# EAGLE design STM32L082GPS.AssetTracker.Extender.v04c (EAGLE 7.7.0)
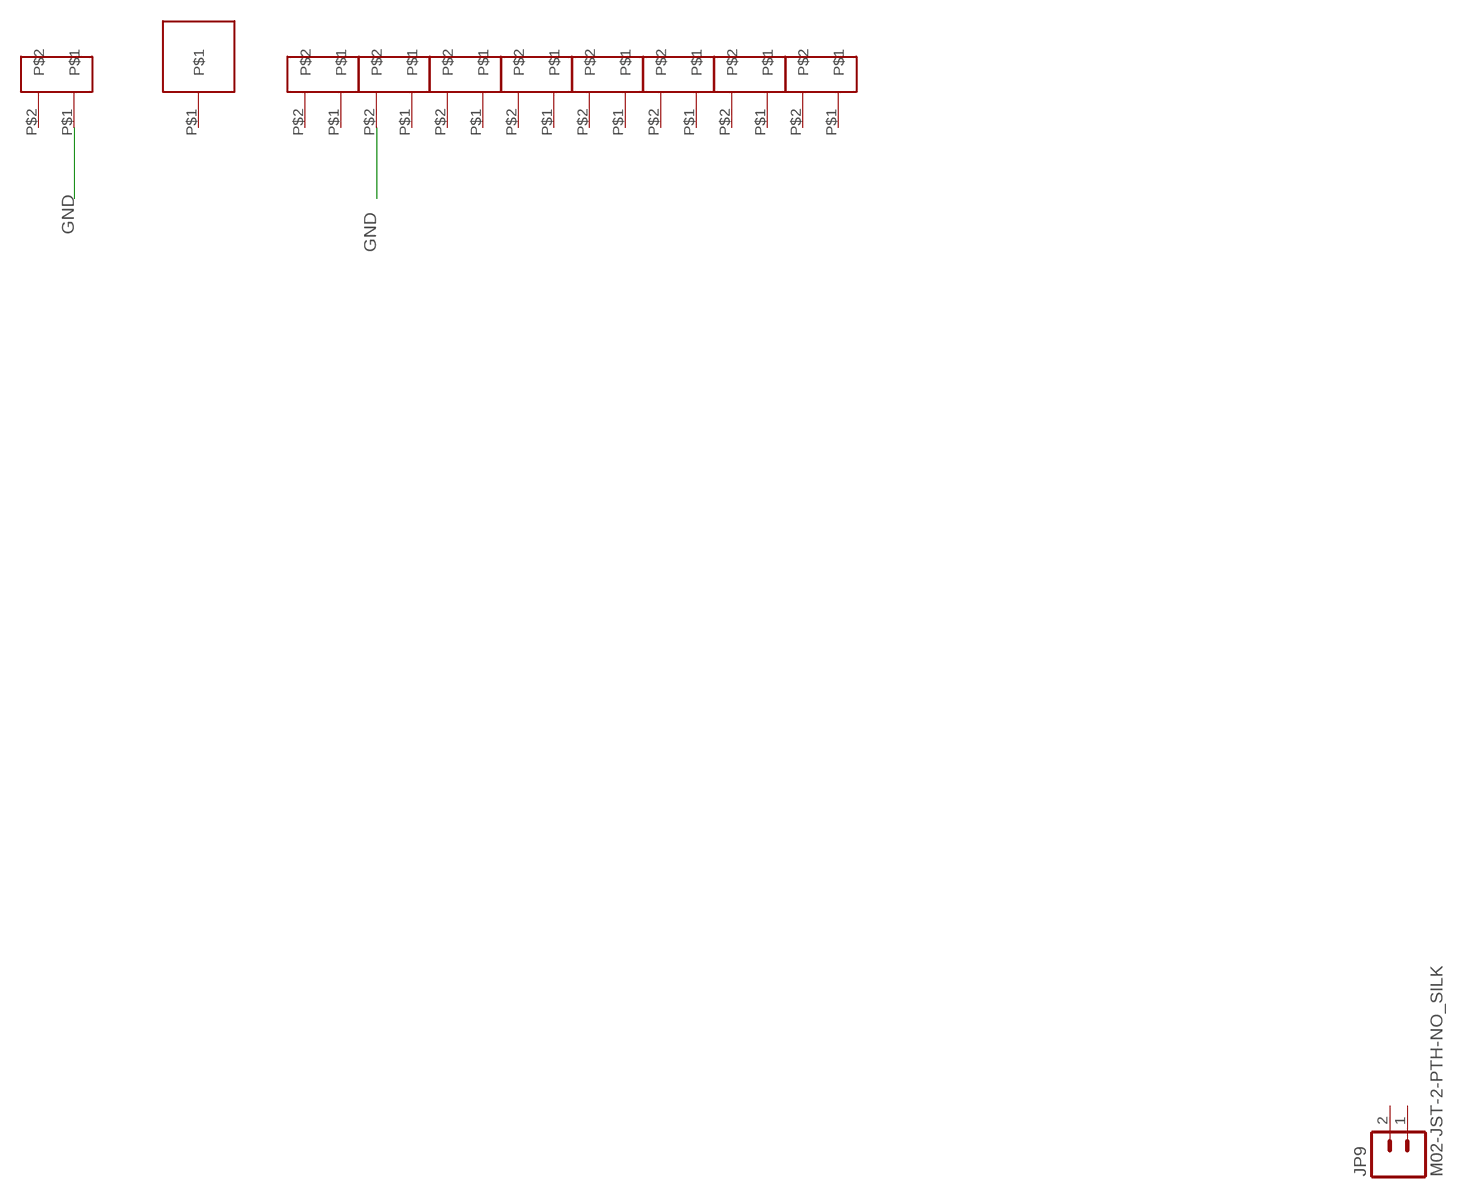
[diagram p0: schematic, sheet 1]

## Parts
JP9  M02-JST-2-PTH-NO_SILK  [JST-2-PTH-NS]
U$1  HN02  [HN02]
U$3  HN02  [HN02]
U$5  HN01  [HN01]
U$11  HN02  [HN02]
U$12  HN02  [HN02]
U$13  HN02  [HN02]
U$14  HN02  [HN02]
U$16  HN02  [HN02]
U$17  HN02  [HN02]
U$36  HN02  [HN02]

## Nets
GND: U$12.P$2 U$36.P$1
Unconnected: JP9.1 JP9.2 U$1.P$1 U$1.P$2 U$3.P$1 U$3.P$2 U$11.P$1 U$11.P$2 U$12.P$1 U$13.P$1 U$13.P$2 U$14.P$1 U$14.P$2 U$16.P$1 U$16.P$2 U$17.P$1 U$17.P$2 U$36.P$2

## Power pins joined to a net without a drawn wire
P$1: U$5.P$1

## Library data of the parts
JP9 = SparkFun-Connectors:M02: Standard 2-pin 0.1" header. Use with
U$1 U$3 U$11-U$14 U$16 U$17 U$36 = Kris:HN02: 0.1 inch header
U$5 = PWSONN6:HN01

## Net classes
1 USB: width 0.254 mm, drill 0.33 mm, clearance 0.159 mm
2 Top GND Pour: clearance 0.762 mm to class 1

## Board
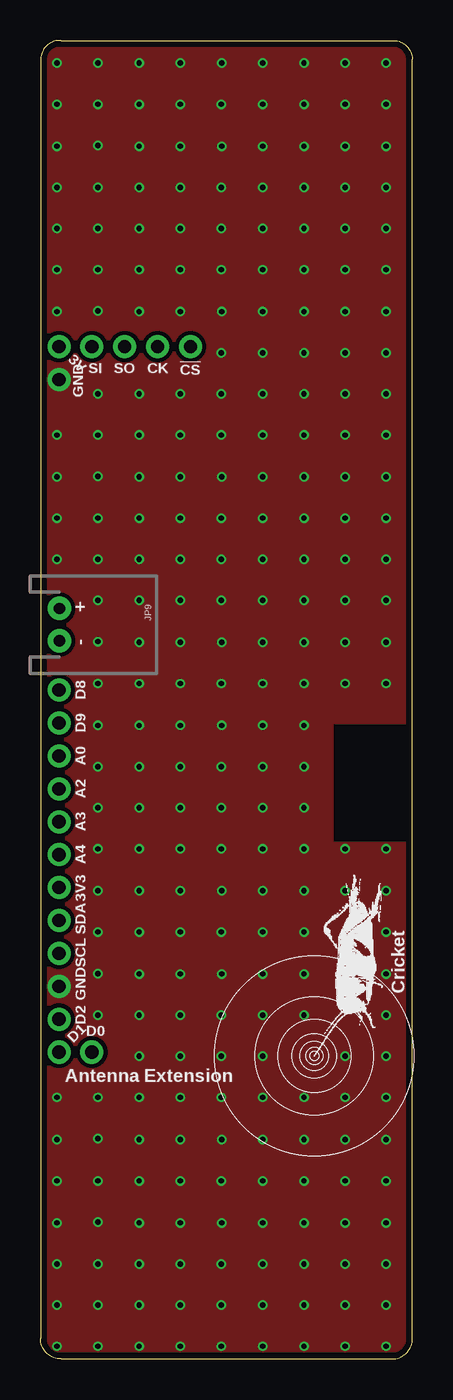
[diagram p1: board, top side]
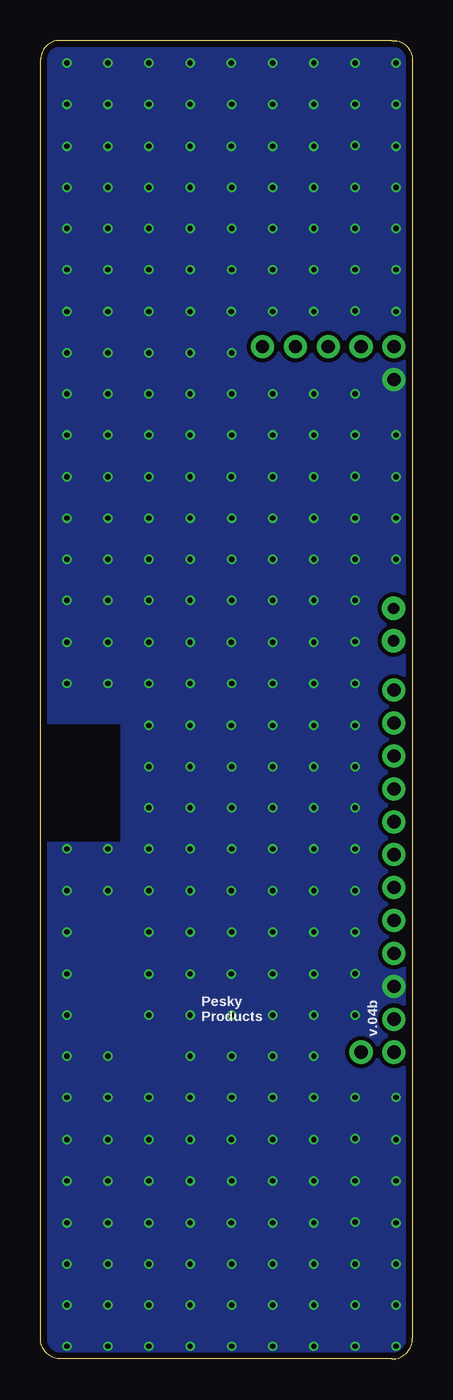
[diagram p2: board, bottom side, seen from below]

Size 22.99 x 81.41 mm. Coordinates in mm from the lower left corner, seen from the top.
Outline: 1.27,0 21.72,0 arc90 22.99,1.27 22.99,80.26 arc90 21.72,81.41 1.27,81.41 arc90 0,80.26 0,1.27 arc90 1.27,0
Copper layers (1*16): Top 0.035559375mm / dielectric 1.6mm / Bottom 0.035559375mm
Design rules "oshpark-2layer *": minimum track width 6mil, minimum drill 10mil, track to track 6mil, track to pad 6mil, pad to pad 6mil, via to via 6mil, smd to smd 6mil, copper to edge 15mil, drill to drill 6mil, minimum pad ring 5mil, minimum via ring 5mil, stop-mask expansion 2.5mil, vias tented up to drill 20mil, thermal gap 10mil

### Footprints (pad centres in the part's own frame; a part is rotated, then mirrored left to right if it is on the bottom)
JST-2-PTH-NS = drill 0.7 pad 1.448: 1 -1,0; 2 1,0
HN02 = drill 0.813 pad 1.422: P$1 0,0; P$2 -2.032,0
HN01 = drill 0.813 pad 1.422: P$1 0,0

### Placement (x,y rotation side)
JP9  1.17,45.34 270 top
U$1  9.27,62.51 0 top
U$3  5.21,62.51 0 top
U$5  1.14,20.98 0 top
U$11  1.14,18.95 180 top
U$12  1.14,25.04 90 top
U$13  1.14,29.11 90 top
U$14  1.14,33.17 90 top
U$16  1.14,41.3 90 top
U$17  1.14,37.24 90 top
U$36  1.14,60.48 270 top

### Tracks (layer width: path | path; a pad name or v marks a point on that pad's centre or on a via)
GND  (via drill 0.33)
  other vias: 1.02,80.01 3.56,80.01 6.1,80.01 8.64,80.01 1.02,77.47 3.56,77.47 6.1,77.47 8.64,77.47 11.18,77.47 3.56,74.93 11.2,80.01 13.74,80.01 16.28,80.01 18.82,80.01 21.36,80.01 13.74,77.47 16.28,77.47 18.82,77.47 21.36,77.47 1.02,74.88 6.1,74.88 8.64,74.88 1.02,72.34 3.56,72.34 6.1,72.34 8.64,72.34 11.18,72.34 1.02,69.8 3.56,69.8 6.1,69.8 8.64,69.8 11.18,69.8 11.2,74.88 13.74,74.88 16.28,74.88 18.82,74.88 21.36,74.88 13.74,72.34 16.28,72.34 18.82,72.34 21.36,72.34 13.74,69.8 16.28,69.8 18.82,69.8 21.36,69.8 1.02,67.26 3.56,67.26 6.1,67.26 8.64,67.26 11.18,67.26 3.56,64.72 13.74,67.26 16.28,67.26 18.82,67.26 21.36,67.26 1.02,64.67 6.1,64.67 8.64,64.67 11.18,62.13 3.56,59.59 6.1,59.59 8.64,59.59 11.18,59.59 11.2,64.67 13.74,64.67 16.28,64.67 18.82,64.67 21.36,64.67 13.74,62.13 16.28,62.13 18.82,62.13 21.36,62.13 13.74,59.59 16.28,59.59 18.82,59.59 21.36,59.59 1.02,57.05 3.56,57.05 6.1,57.05 8.64,57.05 11.18,57.05 3.56,54.51 13.74,57.05 16.28,57.05 18.82,57.05 21.36,57.05 1.02,54.46 6.1,54.46 8.64,54.46 1.02,51.92 3.56,51.92 6.1,51.92 8.64,51.92 11.18,51.92 1.02,49.38 3.56,49.38 6.1,49.38 8.64,49.38 11.18,49.38 11.2,54.46 13.74,54.46 16.28,54.46 18.82,54.46 21.36,54.46 13.74,51.92 16.28,51.92 18.82,51.92 21.36,51.92 13.74,49.38 16.28,49.38 18.82,49.38 21.36,49.38 3.56,46.84 6.1,46.84 8.64,46.84 11.18,46.84 3.56,44.3 13.74,46.84 16.28,46.84 18.82,46.84 21.36,46.84 6.1,44.25 8.64,44.25 11.2,44.25 13.74,44.25 16.28,44.25 18.82,44.25 21.36,44.25 3.56,41.71 6.1,41.71 8.64,41.71 11.18,41.71 3.56,39.12 13.74,41.71 16.28,41.71 18.82,41.71 21.36,41.71 6.1,39.12 8.64,39.12 3.56,36.58 6.1,36.58 8.64,36.58 11.18,36.58 3.56,34.04 6.1,34.04 8.64,34.04 11.18,34.04 11.2,39.12 13.74,39.12 16.28,39.12 13.74,36.58 16.28,36.58 13.74,34.04 16.28,34.04 3.56,31.5 6.1,31.5 8.64,31.5 11.18,31.5 13.74,31.5 16.28,31.5 18.82,31.5 21.36,31.5 6.1,28.91 8.64,28.91 11.2,28.91 13.74,28.91 16.28,28.91 18.82,28.91 21.36,28.91 3.56,28.91 3.56,26.37 6.1,26.37 8.64,26.37 11.18,26.37 3.56,23.8 13.74,26.37 16.28,26.37 21.36,26.37 6.1,23.77 8.64,23.77 3.56,21.23 6.1,21.23 8.64,21.23 11.18,21.23 6.1,18.69 8.64,18.69 11.18,18.69 11.2,23.77 13.74,23.77 16.28,23.77 21.36,23.77 13.74,21.23 16.28,21.23 21.36,21.23 13.74,18.69 18.82,18.69 21.36,18.69 1.02,16.15 3.56,16.15 6.1,16.15 8.64,16.15 11.18,16.15 3.56,13.61 13.74,16.15 16.28,16.15 18.82,16.15 21.36,16.15 1.02,13.54 6.1,13.54 8.64,13.54 1.02,11 3.56,11 6.1,11 8.64,11 11.18,11 3.56,8.46 11.2,13.54 13.74,13.54 16.28,13.54 18.82,13.54 21.36,13.54 13.74,11 16.28,11 18.82,11 21.36,11 1.02,8.41 6.1,8.41 8.64,8.41 1.02,5.87 3.56,5.87 6.1,5.87 8.64,5.87 11.18,5.87 1.02,3.33 3.56,3.33 6.1,3.33 8.64,3.33 11.18,3.33 11.2,8.41 13.74,8.41 16.28,8.41 18.82,8.41 21.36,8.41 13.74,5.87 16.28,5.87 18.82,5.87 21.36,5.87 13.74,3.33 16.28,3.33 18.82,3.33 21.36,3.33 1.02,0.79 3.56,0.79 6.1,0.79 8.64,0.79 11.18,0.79 13.74,0.79 16.28,0.79 18.82,0.79 21.36,0.79
  pour Top (isolate 0.254, no thermals): 0,0 0,81.41 22.99,81.41 23.06,39.29 17.98,39.29 17.98,31.83 22.96,31.83 22.96,0
  pour Bottom (isolate 0.254, no thermals): 0,0 22.99,0 22.99,81.41 0,81.41 -0.03,58.65 0,58.65
N$2
  cutout Bottom (isolate 0.254): 23.04,39.17 18.11,39.17 18.11,31.95 23.04,31.95

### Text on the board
tPlace: 3V | SI | SO | CK | !CS | GND | + | - | D8 | D9 | A0 | A2 | A3 | A4 | 3V3 | SDA | SCL | Cricket | GND | D2 | D0 | D1 | Antenna Extension
bPlace: Pesky / Products | v.04b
